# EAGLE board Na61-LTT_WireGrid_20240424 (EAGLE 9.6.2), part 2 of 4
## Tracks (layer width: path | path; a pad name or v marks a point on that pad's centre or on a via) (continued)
S$1547 (continued)
  Bottom 0.152: 49.8,31 49.4,31
S$1548
  Bottom 0.152: 49.4,31 48.4,32
S$1549
  Bottom 0.152: 47.8,31 46.8,32
S$1550
  Bottom 0.152: 45.8,31 45.2,31.6
S$1551
  Bottom 0.152: 45.2,31.6 45.2,32
S$1552
  Bottom 0.152: 43.8,31 43.6,31.2
S$1553
  Bottom 0.152: 43.6,31.2 43.6,32
S$1554
  Bottom 0.152: 41.8,31 42,31.2
S$1555
  Bottom 0.152: 42,31.2 42,32
S$1556
  Bottom 0.152: 39.8,31 40.4,31.6
S$1557
  Bottom 0.152: 40.4,31.6 40.4,32
S$1558
  Bottom 0.152: 37.8,31 38.8,32
S$1559
  Bottom 0.152: 35.8,31 36.2,31
S$1560
  Bottom 0.152: 36.2,31 37.2,32
S$1561
  Bottom 0.152: 33.8,31 34.6,31
S$1562
  Bottom 0.152: 34.6,31 35.6,32
S$1563
  Bottom 0.152: 40.8,35 41.2,35.4
S$1564
  Bottom 0.152: 41.2,35.4 41.2,36
S$1565
  Bottom 0.152: 38.8,35 39.6,35.8
S$1566
  Bottom 0.152: 39.6,35.8 39.6,36
S$1567
  Bottom 0.152: 36.8,35 37,35
S$1568
  Bottom 0.152: 37,35 38,36
S$1569
  Bottom 0.152: 34.8,35 35.4,35
S$1570
  Bottom 0.152: 35.4,35 36.4,36
S$1571
  Bottom 0.152: 32.8,33 33.8,32
S$1572
  Bottom 0.152: 33.8,32 34.8,32
S$1573
  Bottom 0.152: 34.6,37 34,37
S$1574
  Bottom 0.152: 34,37 33,36
S$1575
  Bottom 0.152: 33,36 32.4,36
S$1576
  Bottom 0.152: 32.6,37 31.6,36
S$1577
  Bottom 0.152: 31.6,36 30.8,36
S$1578
  Bottom 0.152: 30.6,37 29.6,36
S$1579
  Bottom 0.152: 29.6,36 29.2,36
S$1580
  Bottom 0.152: 28.6,37 27.6,36
S$1581
  Bottom 0.152: 26.6,37 26,36.4
S$1582
  Bottom 0.152: 26,36.4 26,36
S$1583
  Bottom 0.152: 35.6,41 34.6,40
S$1584
  Bottom 0.152: 34.6,40 33.2,40
S$1585
  Bottom 0.152: 33.6,41 33.2,41
S$1586
  Bottom 0.152: 33.2,41 32.2,40
S$1587
  Bottom 0.152: 32.2,40 31.6,40
S$1588
  Bottom 0.152: 31.6,41 31,41
S$1589
  Bottom 0.152: 31,41 30,40
S$1590
  Bottom 0.152: 29.6,41 29.4,41
S$1591
  Bottom 0.152: 29.4,41 28.4,40
S$1592
  Bottom 0.152: 27.6,41 26.8,40.2
S$1593
  Bottom 0.152: 26.8,40.2 26.8,40
S$1594
  Bottom 0.152: 34,36 35.2,36
S$1595
  Bottom 0.152: 35.2,36 36.2,37
S$1596
  Bottom 0.152: 36.2,37 36.6,37
S$1597  (2 unrouted)
  Top 0.813: 65,40.5 65,31.5
  Top 1.8: 66,37.5 64,37.5 | 66,40.5 65,40.5 64,40.5 | 66,34.5 64,34.5 | 66,31.5 65,31.5 64,31.5
S$1598
  Top 1.778: -104.08,32.83 -104.08,34.35
S$1599
  Top 1.778: -104.08,37.65 -104.08,39.17
S$1600
  Top 1.778: -99,32.83 -99,34.35
S$1601
  Top 1.778: -99,37.65 -99,39.17
S$1602
  Top 1.778: -93.92,32.83 -93.92,34.35
S$1603
  Top 1.778: -93.92,37.65 -93.92,39.17
S$1604
  Top 1.778: 93.92,32.83 93.92,34.35
S$1605
  Top 1.778: 93.92,37.65 93.92,39.17
S$1606
  Top 1.778: 99,32.83 99,34.35
S$1607
  Top 1.778: 99,37.65 99,39.17
S$1608
  Top 1.778: 104.08,32.83 104.08,34.35
S$1609
  Top 1.778: 104.08,37.65 104.08,39.17
S$1618
  Bottom 0.8: 9.4,48.9 9.4,47.1
S$1619
  Bottom 0.8: 11.4,48.9 11.4,47.1
S$1620
  Bottom 0.8: 8.4,51.1 8.4,52.9
S$1621
  Bottom 0.8: 10.4,51.1 10.4,52.9
S$1622
  Bottom 0.8: 5.4,48.9 5.4,47.1
S$1623
  Bottom 0.8: 7.4,48.9 7.4,47.1
S$1624
  Bottom 0.8: 6.4,51.1 6.4,52.9
S$1625
  Bottom 0.8: 4.4,51.1 4.4,52.9
S$1626
  Bottom 0.8: 3.4,48.9 3.4,47.1
S$1627
  Bottom 0.8: 1.4,48.9 1.4,47.1
S$1628
  Bottom 0.8: 2.4,51.1 2.4,52.9
S$1629
  Bottom 0.8: 0.4,51.1 0.4,52.9
S$1630
  Bottom 0.8: -0.6,48.9 -0.6,47.1
S$1631
  Bottom 0.8: -2.6,48.9 -2.6,47.1
S$1632
  Bottom 0.8: -1.6,51.1 -1.6,52.9
S$1633
  Bottom 0.8: 17.4,48.9 17.4,47.1
S$1634
  Bottom 0.8: 19.4,48.9 19.4,47.1
S$1635
  Bottom 0.8: 16.4,51.1 16.4,52.9
S$1636
  Bottom 0.8: 18.4,51.1 18.4,52.9
S$1637
  Bottom 0.8: 13.4,48.9 13.4,47.1
S$1638
  Bottom 0.8: 15.4,48.9 15.4,47.1
S$1639
  Bottom 0.8: 12.4,51.1 12.4,52.9
S$1640
  Bottom 0.8: 14.4,51.1 14.4,52.9
S$1641
  Bottom 0.8: -7.4,56.9 -7.4,55.1
S$1642
  Bottom 0.8: -5.4,56.9 -5.4,55.1
S$1643
  Bottom 0.8: -8.4,59.1 -8.4,60.9
S$1644
  Bottom 0.8: -6.4,59.1 -6.4,60.9
S$1645
  Bottom 0.8: -11.4,56.9 -11.4,55.1
S$1646
  Bottom 0.8: -9.4,56.9 -9.4,55.1
S$1647
  Bottom 0.8: -10.4,59.1 -10.4,60.9
S$1648
  Bottom 0.8: -12.4,59.1 -12.4,60.9
S$1649
  Bottom 0.8: -13.4,56.9 -13.4,55.1
S$1650
  Bottom 0.8: -15.4,56.9 -15.4,55.1
S$1651
  Bottom 0.8: -14.4,59.1 -14.4,60.9
S$1652
  Bottom 0.8: -16.4,59.1 -16.4,60.9
S$1653
  Bottom 0.8: -17.4,56.9 -17.4,55.1
S$1654
  Bottom 0.8: -19.4,56.9 -19.4,55.1
S$1655
  Bottom 0.8: -18.4,59.1 -18.4,60.9
S$1656
  Bottom 0.8: 0.6,56.9 0.6,55.1
S$1657
  Bottom 0.8: 2.6,56.9 2.6,55.1
S$1658
  Bottom 0.8: -0.4,59.1 -0.4,60.9
S$1659
  Bottom 0.8: 1.6,59.1 1.6,60.9
S$1660
  Bottom 0.8: -3.4,56.9 -3.4,55.1
S$1661
  Bottom 0.8: -1.4,56.9 -1.4,55.1
S$1662
  Bottom 0.8: -4.4,59.1 -4.4,60.9
S$1663
  Bottom 0.8: -2.4,59.1 -2.4,60.9
S$1664
  Bottom 0.8: -24.6,48.9 -24.6,47.1
S$1665
  Bottom 0.8: -22.6,48.9 -22.6,47.1
S$1666
  Bottom 0.8: -25.6,51.1 -25.6,52.9
S$1667
  Bottom 0.8: -23.6,51.1 -23.6,52.9
S$1668
  Bottom 0.8: -28.6,48.9 -28.6,47.1
S$1669
  Bottom 0.8: -26.6,48.9 -26.6,47.1
S$1670
  Bottom 0.8: -27.6,51.1 -27.6,52.9
S$1671
  Bottom 0.8: -29.6,51.1 -29.6,52.9
S$1672
  Bottom 0.8: -30.6,48.9 -30.6,47.1
S$1673
  Bottom 0.8: -32.6,48.9 -32.6,47.1
S$1674
  Bottom 0.8: -31.6,51.1 -31.6,52.9
S$1675
  Bottom 0.8: -33.6,51.1 -33.6,52.9
S$1676
  Bottom 0.8: -34.6,48.9 -34.6,47.1
S$1677
  Bottom 0.8: -36.6,48.9 -36.6,47.1
S$1678
  Bottom 0.8: -35.6,51.1 -35.6,52.9
S$1679
  Bottom 0.8: -16.6,48.9 -16.6,47.1
S$1680
  Bottom 0.8: -14.6,48.9 -14.6,47.1
S$1681
  Bottom 0.8: -17.6,51.1 -17.6,52.9
S$1682
  Bottom 0.8: -15.6,51.1 -15.6,52.9
S$1683
  Bottom 0.8: -20.6,48.9 -20.6,47.1
S$1684
  Bottom 0.8: -18.6,48.9 -18.6,47.1
S$1685
  Bottom 0.8: -21.6,51.1 -21.6,52.9
S$1686
  Bottom 0.8: -19.6,51.1 -19.6,52.9
S$1687
  Bottom 0.8: 26.6,56.9 26.6,55.1
S$1688
  Bottom 0.8: 28.6,56.9 28.6,55.1
S$1689
  Bottom 0.8: 25.6,59.1 25.6,60.9
S$1690
  Bottom 0.8: 27.6,59.1 27.6,60.9
S$1691
  Bottom 0.8: 22.6,56.9 22.6,55.1
S$1692
  Bottom 0.8: 24.6,56.9 24.6,55.1
S$1693
  Bottom 0.8: 23.6,59.1 23.6,60.9
S$1694
  Bottom 0.8: 21.6,59.1 21.6,60.9
S$1695
  Bottom 0.8: 20.6,56.9 20.6,55.1
S$1696
  Bottom 0.8: 18.6,56.9 18.6,55.1
S$1697
  Bottom 0.8: 19.6,59.1 19.6,60.9
S$1698
  Bottom 0.8: 17.6,59.1 17.6,60.9
S$1699
  Bottom 0.8: 16.6,56.9 16.6,55.1
S$1700
  Bottom 0.8: 14.6,56.9 14.6,55.1
S$1701
  Bottom 0.8: 15.6,59.1 15.6,60.9
S$1702
  Bottom 0.8: 34.6,56.9 34.6,55.1
S$1703
  Bottom 0.8: 36.6,56.9 36.6,55.1
S$1704
  Bottom 0.8: 33.6,59.1 33.6,60.9
S$1705
  Bottom 0.8: 35.6,59.1 35.6,60.9
S$1706
  Bottom 0.8: 30.6,56.9 30.6,55.1
S$1707
  Bottom 0.8: 32.6,56.9 32.6,55.1
S$1708
  Bottom 0.8: 29.6,59.1 29.6,60.9
S$1709
  Bottom 0.8: 31.6,59.1 31.6,60.9
S$1710
  Bottom 0.8: -41.8,56.9 -41.8,55.1
S$1711
  Bottom 0.8: -39.8,56.9 -39.8,55.1
S$1712
  Bottom 0.8: -42.8,59.1 -42.8,60.9
S$1713
  Bottom 0.8: -40.8,59.1 -40.8,60.9
S$1714
  Bottom 0.8: -45.8,56.9 -45.8,55.1
S$1715
  Bottom 0.8: -43.8,56.9 -43.8,55.1
S$1716
  Bottom 0.8: -44.8,59.1 -44.8,60.9
S$1717
  Bottom 0.8: -46.8,59.1 -46.8,60.9
S$1718
  Bottom 0.8: -47.8,56.9 -47.8,55.1
S$1719
  Bottom 0.8: -49.8,56.9 -49.8,55.1
S$1720
  Bottom 0.8: -48.8,59.1 -48.8,60.9
S$1721
  Bottom 0.8: -50.8,59.1 -50.8,60.9
S$1722
  Bottom 0.8: -51.8,56.9 -51.8,55.1
S$1723
  Bottom 0.8: -53.8,56.9 -53.8,55.1
S$1724
  Bottom 0.8: -52.8,59.1 -52.8,60.9
S$1725
  Bottom 0.8: -33.8,56.9 -33.8,55.1
S$1726
  Bottom 0.8: -31.8,56.9 -31.8,55.1
S$1727
  Bottom 0.8: -34.8,59.1 -34.8,60.9
S$1728
  Bottom 0.8: -32.8,59.1 -32.8,60.9
S$1729
  Bottom 0.8: -37.8,56.9 -37.8,55.1
S$1730
  Bottom 0.8: -35.8,56.9 -35.8,55.1
S$1731
  Bottom 0.8: -38.8,59.1 -38.8,60.9
S$1732
  Bottom 0.8: -36.8,59.1 -36.8,60.9
S$1733
  Bottom 0.8: 43.8,48.9 43.8,47.1
S$1734
  Bottom 0.8: 45.8,48.9 45.8,47.1
S$1735
  Bottom 0.8: 42.8,51.1 42.8,52.9
S$1736
  Bottom 0.8: 44.8,51.1 44.8,52.9
S$1737
  Bottom 0.8: 39.8,48.9 39.8,47.1
S$1738
  Bottom 0.8: 41.8,48.9 41.8,47.1
S$1739
  Bottom 0.8: 40.8,51.1 40.8,52.9
S$1740
  Bottom 0.8: 38.8,51.1 38.8,52.9
S$1741
  Bottom 0.8: 37.8,48.9 37.8,47.1
S$1742
  Bottom 0.8: 35.8,48.9 35.8,47.1
S$1743
  Bottom 0.8: 36.8,51.1 36.8,52.9
S$1744
  Bottom 0.8: 34.8,51.1 34.8,52.9
S$1745
  Bottom 0.8: 33.8,48.9 33.8,47.1
S$1746
  Bottom 0.8: 31.8,48.9 31.8,47.1
S$1747
  Bottom 0.8: 32.8,51.1 32.8,52.9
S$1748
  Bottom 0.8: 51.8,48.9 51.8,47.1
S$1749
  Bottom 0.8: 53.8,48.9 53.8,47.1
S$1750
  Bottom 0.8: 50.8,51.1 50.8,52.9
S$1751
  Bottom 0.8: 52.8,51.1 52.8,52.9
S$1752
  Bottom 0.8: 47.8,48.9 47.8,47.1
S$1753
  Bottom 0.8: 49.8,48.9 49.8,47.1
S$1754
  Bottom 0.8: 46.8,51.1 46.8,52.9
S$1755
  Bottom 0.8: 48.8,51.1 48.8,52.9
S$1884
  Bottom 0.152: -52.8,59 -51.8,58
S$1885
  Bottom 0.152: -51.8,58 -50.8,58
S$1886
  Bottom 0.152: -50.8,59 -50.2,59
S$1887
  Bottom 0.152: -50.2,59 -49.2,58
S$1888
  Bottom 0.152: -48.8,59 -48.6,59
S$1889
  Bottom 0.152: -48.6,59 -47.6,58
S$1890
  Bottom 0.152: -46.8,59 -46,58.2
S$1891
  Bottom 0.152: -46,58.2 -46,58
S$1892
  Bottom 0.152: -44.8,59 -44.4,58.6
S$1893
  Bottom 0.152: -44.4,58.6 -44.4,58
S$1894
  Bottom 0.152: -42.8,59 -42.8,58
S$1895
  Bottom 0.152: -40.8,59 -41.2,58.6
S$1896
  Bottom 0.152: -41.2,58.6 -41.2,58
S$1897
  Bottom 0.152: -38.8,59 -39.6,58.2
S$1898
  Bottom 0.152: -39.6,58.2 -39.6,58
S$1899
  Bottom 0.152: -36.8,59 -37,59
S$1900
  Bottom 0.152: -37,59 -38,58
S$1901
  Bottom 0.152: -34.8,59 -35.4,59
S$1902
  Bottom 0.152: -35.4,59 -36.4,58
S$1903
  Bottom 0.152: -32.8,59 -33.8,58
S$1904
  Bottom 0.152: -33.8,58 -34.8,58
S$1905
  Bottom 0.152: -51.8,55 -50.8,54
S$1906
  Bottom 0.152: -50.8,54 -50,54
S$1907
  Bottom 0.152: -49.8,55 -48.8,54
S$1908
  Bottom 0.152: -48.8,54 -48.4,54
S$1909
  Bottom 0.152: -47.8,55 -46.8,54
S$1910
  Bottom 0.152: -45.8,55 -45.2,54.4
S$1911
  Bottom 0.152: -45.2,54.4 -45.2,54
S$1912
  Bottom 0.152: -43.8,55 -43.6,54.8
S$1913
  Bottom 0.152: -43.6,54.8 -43.6,54
S$1914
  Bottom 0.152: -41.8,55 -42,54.8
S$1915
  Bottom 0.152: -42,54.8 -42,54
S$1916
  Bottom 0.152: -39.8,55 -40.4,54.4
S$1917
  Bottom 0.152: -40.4,54.4 -40.4,54
S$1918
  Bottom 0.152: -37.8,55 -38.8,54
S$1919
  Bottom 0.152: -35.8,55 -36.8,54
S$1920
  Bottom 0.152: -36.8,54 -37.2,54
S$1921
  Bottom 0.152: -33.8,55 -34.8,54
S$1922
  Bottom 0.152: -34.8,54 -35.6,54
S$1923
  Bottom 0.152: -36.6,49 -35.6,50
S$1924
  Bottom 0.152: -35.6,50 -34,50
S$1925
  Bottom 0.152: -34.6,49 -33.8,49
S$1926
  Bottom 0.152: -33.8,49 -32.8,50
S$1927
  Bottom 0.152: -32.8,50 -32.4,50
S$1928
  Bottom 0.152: -32.6,49 -31.8,49
S$1929
  Bottom 0.152: -31.8,49 -30.8,50
S$1930
  Bottom 0.152: -30.6,49 -30.2,49
S$1931
  Bottom 0.152: -30.2,49 -29.2,50
S$1932
  Bottom 0.152: -28.6,49 -27.6,50
S$1933
  Bottom 0.152: -26.6,49 -26,49.6
S$1934
  Bottom 0.152: -26,49.6 -26,50
S$1935
  Bottom 0.152: -35.6,53 -35,53
S$1936
  Bottom 0.152: -35,53 -34,54
S$1937
  Bottom 0.152: -34,54 -33.2,54
S$1938
  Bottom 0.152: -33.6,53 -33,53
S$1939
  Bottom 0.152: -33,53 -32,54
S$1940
  Bottom 0.152: -32,54 -31.6,54
S$1941
  Bottom 0.152: -31.6,53 -31,53
S$1942
  Bottom 0.152: -31,53 -30,54
S$1943
  Bottom 0.152: -29.6,53 -29.4,53
S$1944
  Bottom 0.152: -29.4,53 -28.4,54
S$1945
  Bottom 0.152: -27.6,53 -26.8,53.8
S$1946
  Bottom 0.152: -26.8,53.8 -26.8,54
S$1947
  Bottom 0.152: 1.6,59 0.6,58
S$1948
  Bottom 0.152: 0.6,58 -0.4,58
S$1949
  Bottom 0.152: -0.4,59 -1,59
S$1950
  Bottom 0.152: -1,59 -2,58
S$1951
  Bottom 0.152: -2.4,59 -2.6,59
S$1952
  Bottom 0.152: -2.6,59 -3.6,58
S$1953
  Bottom 0.152: -4.4,59 -5.2,58.2
S$1954
  Bottom 0.152: -5.2,58.2 -5.2,58
S$1955
  Bottom 0.152: -6.4,59 -6.8,58.6
S$1956
  Bottom 0.152: -6.8,58.6 -6.8,58
S$1957
  Bottom 0.152: -8.4,59 -8.4,58
S$1958
  Bottom 0.152: -10.4,59 -10,58.6
S$1959
  Bottom 0.152: -10,58.6 -10,58
S$1960
  Bottom 0.152: -12.4,59 -11.6,58.2
S$1961
  Bottom 0.152: -11.6,58.2 -11.6,58
S$1962
  Bottom 0.152: -14.4,59 -14.2,59
S$1963
  Bottom 0.152: -14.2,59 -13.2,58
S$1964
  Bottom 0.152: -16.4,59 -15.8,59
S$1965
  Bottom 0.152: -15.8,59 -14.8,58
S$1966
  Bottom 0.152: -18.4,59 -17.4,58
S$1967
  Bottom 0.152: -17.4,58 -16.4,58
S$1968
  Bottom 0.152: 0.6,55 -0.4,54
S$1969
  Bottom 0.152: -0.4,54 -1.2,54
S$1970
  Bottom 0.152: -1.4,55 -2.4,54
S$1971
  Bottom 0.152: -2.4,54 -2.8,54
S$1972
  Bottom 0.152: -3.4,55 -4.4,54
S$1973
  Bottom 0.152: -5.4,55 -6,54.4
S$1974
  Bottom 0.152: -6,54.4 -6,54
S$1975
  Bottom 0.152: -7.4,55 -7.6,54.8
S$1976
  Bottom 0.152: -7.6,54.8 -7.6,54
S$1977
  Bottom 0.152: -9.4,55 -9.2,54.8
S$1978
  Bottom 0.152: -9.2,54.8 -9.2,54
S$1979
  Bottom 0.152: -11.4,55 -10.8,54.4
S$1980
  Bottom 0.152: -10.8,54.4 -10.8,54
S$1981
  Bottom 0.152: -13.4,55 -12.4,54
S$1982
  Bottom 0.152: -15.4,55 -14.4,54
S$1983
  Bottom 0.152: -14.4,54 -14,54
S$1984
  Bottom 0.152: -17.4,55 -16.4,54
S$1985
  Bottom 0.152: -16.4,54 -15.6,54
S$1986
  Bottom 0.152: -14.6,49 -15.6,50
S$1987
  Bottom 0.152: -15.6,50 -17.2,50
S$1988
  Bottom 0.152: -16.6,49 -17.4,49
S$1989
  Bottom 0.152: -17.4,49 -18.4,50
S$1990
  Bottom 0.152: -18.4,50 -18.8,50
S$1991
  Bottom 0.152: -18.6,49 -19.4,49
S$1992
  Bottom 0.152: -19.4,49 -20.4,50
S$1993
  Bottom 0.152: -20.6,49 -21,49
S$1994
  Bottom 0.152: -21,49 -22,50
S$1995
  Bottom 0.152: -22.6,49 -23.6,50
S$1996
  Bottom 0.152: -24.6,49 -25.2,49.6
S$1997
  Bottom 0.152: -25.2,49.6 -25.2,50
S$1998
  Bottom 0.152: -15.6,53 -16.2,53
S$1999
  Bottom 0.152: -16.2,53 -17.2,54
S$2000
  Bottom 0.152: -17.2,54 -18,54
S$2001
  Bottom 0.152: -17.6,53 -18.2,53
S$2002
  Bottom 0.152: -18.2,53 -19.2,54
S$2003
  Bottom 0.152: -19.2,54 -19.6,54
S$2004
  Bottom 0.152: -19.6,53 -20.2,53
S$2005
  Bottom 0.152: -20.2,53 -21.2,54
S$2006
  Bottom 0.152: -21.6,53 -21.8,53
S$2007
  Bottom 0.152: -21.8,53 -22.8,54
S$2008
  Bottom 0.152: -23.6,53 -24.4,53.8
S$2009
  Bottom 0.152: -24.4,53.8 -24.4,54
S$2010
  Bottom 0.152: 0.4,53 1,53
S$2011
  Bottom 0.152: 1,53 2,54
S$2012
  Bottom 0.152: 2.4,53 2.6,53
S$2013
  Bottom 0.152: 2.6,53 3.6,54
S$2014
  Bottom 0.152: 4.4,53 5.2,53.8
S$2015
  Bottom 0.152: 5.2,53.8 5.2,54
S$2016
  Bottom 0.152: 6.4,53 6.8,53.4
S$2017
  Bottom 0.152: 6.8,53.4 6.8,54
S$2018
  Bottom 0.152: 8.4,53 8.4,54
S$2019
  Bottom 0.152: -1.6,53 -0.6,53
S$2020
  Bottom 0.152: -0.6,53 0.4,54
S$2021
  Bottom 0.152: -0.6,49 0.4,50
S$2022
  Bottom 0.152: 0.4,50 1.2,50
S$2023
  Bottom 0.152: 1.4,49 1.8,49
S$2024
  Bottom 0.152: 1.8,49 2.8,50
S$2025
  Bottom 0.152: 3.4,49 4.4,50
S$2026
  Bottom 0.152: 5.4,49 6,49.6
S$2027
  Bottom 0.152: 6,49.6 6,50
S$2028
  Bottom 0.152: 7.4,49 7.6,49.2
S$2029
  Bottom 0.152: 7.6,49.2 7.6,50
S$2030
  Bottom 0.152: 9.4,49 9.2,49.2
S$2031
  Bottom 0.152: 9.2,49.2 9.2,50
S$2032
  Bottom 0.152: 11.4,49 10.8,49.6
S$2033
  Bottom 0.152: 10.8,49.6 10.8,50
S$2034
  Bottom 0.152: 13.4,49 12.4,50
S$2035
  Bottom 0.152: 15.4,49 15,49
S$2036
  Bottom 0.152: 15,49 14,50
S$2037
  Bottom 0.152: 17.4,49 16.6,49
S$2038
  Bottom 0.152: 16.6,49 15.6,50
S$2039
  Bottom 0.152: 10.4,53 10,53.4
S$2040
  Bottom 0.152: 10,53.4 10,54
S$2041
  Bottom 0.152: 12.4,53 11.6,53.8
S$2042
  Bottom 0.152: 11.6,53.8 11.6,54
S$2043
  Bottom 0.152: 14.4,53 14.2,53
S$2044
  Bottom 0.152: 14.2,53 13.2,54
S$2045
  Bottom 0.152: 16.4,53 15.8,53
S$2046
  Bottom 0.152: 15.8,53 14.8,54
S$2047
  Bottom 0.152: 18.4,51 17.4,50
S$2048
  Bottom 0.152: 17.4,50 16.4,50
S$2049
  Bottom 0.152: 16.6,55 17.2,55
S$2050
  Bottom 0.152: 17.2,55 18.2,54
S$2051
  Bottom 0.152: 18.2,54 18.8,54
S$2052
  Bottom 0.152: 18.6,55 19.6,54
S$2053
  Bottom 0.152: 19.6,54 20.4,54
S$2054
  Bottom 0.152: 20.6,55 21.6,54
S$2055
  Bottom 0.152: 21.6,54 22,54
S$2056
  Bottom 0.152: 22.6,55 23.6,54
S$2057
  Bottom 0.152: 24.6,55 25.2,54.4
S$2058
  Bottom 0.152: 25.2,54.4 25.2,54
S$2059
  Bottom 0.152: 15.6,59 16.6,58
S$2060
  Bottom 0.152: 16.6,58 18,58
S$2061
  Bottom 0.152: 17.6,59 18,59
S$2062
  Bottom 0.152: 18,59 19,58
S$2063
  Bottom 0.152: 19,58 19.6,58
S$2064
  Bottom 0.152: 19.6,59 20.2,59
S$2065
  Bottom 0.152: 20.2,59 21.2,58
S$2066
  Bottom 0.152: 21.6,59 21.8,59
S$2067
  Bottom 0.152: 21.8,59 22.8,58
S$2068
  Bottom 0.152: 23.6,59 24.4,58.2
S$2069
  Bottom 0.152: 24.4,58.2 24.4,58
S$2070
  Bottom 0.152: 17.2,54 16,54
S$2071
  Bottom 0.152: 16,54 15,55
S$2072
  Bottom 0.152: 15,55 14.6,55
S$2073
  Bottom 0.152: 50.8,53 50.2,53
S$2074
  Bottom 0.152: 50.2,53 49.2,54
S$2075
  Bottom 0.152: 48.8,53 48.6,53
S$2076
  Bottom 0.152: 48.6,53 47.6,54
S$2077
  Bottom 0.152: 46.8,53 46,53.8
S$2078
  Bottom 0.152: 46,53.8 46,54
S$2079
  Bottom 0.152: 44.8,53 44.4,53.4
S$2080
  Bottom 0.152: 44.4,53.4 44.4,54
S$2081
  Bottom 0.152: 42.8,53 42.8,54
S$2082
  Bottom 0.152: 52.8,53 51.8,53
S$2083
  Bottom 0.152: 51.8,53 50.8,54
S$2084
  Bottom 0.152: 51.8,49 50.8,50
S$2085
  Bottom 0.152: 50.8,50 50,50
S$2086
  Bottom 0.152: 49.8,49 49.4,49
S$2087
  Bottom 0.152: 49.4,49 48.4,50
S$2088
  Bottom 0.152: 47.8,49 46.8,50
S$2089
  Bottom 0.152: 45.8,49 45.2,49.6
S$2090
  Bottom 0.152: 45.2,49.6 45.2,50
S$2091
  Bottom 0.152: 43.8,49 43.6,49.2
S$2092
  Bottom 0.152: 43.6,49.2 43.6,50
S$2093
  Bottom 0.152: 41.8,49 42,49.2
S$2094
  Bottom 0.152: 42,49.2 42,50
S$2095
  Bottom 0.152: 39.8,49 40.4,49.6
S$2096
  Bottom 0.152: 40.4,49.6 40.4,50
S$2097
  Bottom 0.152: 37.8,49 38.8,50
S$2098
  Bottom 0.152: 35.8,49 36.2,49
S$2099
  Bottom 0.152: 36.2,49 37.2,50
S$2100
  Bottom 0.152: 33.8,49 34.6,49
S$2101
  Bottom 0.152: 34.6,49 35.6,50
S$2102
  Bottom 0.152: 40.8,53 41.2,53.4
S$2103
  Bottom 0.152: 41.2,53.4 41.2,54
S$2104
  Bottom 0.152: 38.8,53 39.6,53.8
S$2105
  Bottom 0.152: 39.6,53.8 39.6,54
S$2106
  Bottom 0.152: 36.8,53 37,53
S$2107
  Bottom 0.152: 37,53 38,54
S$2108
  Bottom 0.152: 34.8,53 35.4,53
S$2109
  Bottom 0.152: 35.4,53 36.4,54
S$2110
  Bottom 0.152: 32.8,51 33.8,50
S$2111
  Bottom 0.152: 33.8,50 34.8,50
S$2112
  Bottom 0.152: 34.6,55 34,55
S$2113
  Bottom 0.152: 34,55 33,54
S$2114
  Bottom 0.152: 33,54 32.4,54
S$2115
  Bottom 0.152: 32.6,55 31.6,54
S$2116
  Bottom 0.152: 31.6,54 30.8,54
S$2117
  Bottom 0.152: 30.6,55 29.6,54
S$2118
  Bottom 0.152: 29.6,54 29.2,54
S$2119
  Bottom 0.152: 28.6,55 27.6,54
S$2120
  Bottom 0.152: 26.6,55 26,54.4
S$2121
  Bottom 0.152: 26,54.4 26,54
S$2122
  Bottom 0.152: 35.6,59 34.6,58
S$2123
  Bottom 0.152: 34.6,58 33.2,58
S$2124
  Bottom 0.152: 33.6,59 33.2,59
S$2125
  Bottom 0.152: 33.2,59 32.2,58
S$2126
  Bottom 0.152: 32.2,58 31.6,58
S$2127
  Bottom 0.152: 31.6,59 31,59
S$2128
  Bottom 0.152: 31,59 30,58
S$2129
  Bottom 0.152: 29.6,59 29.4,59
S$2130
  Bottom 0.152: 29.4,59 28.4,58
S$2131
  Bottom 0.152: 27.6,59 26.8,58.2
S$2132
  Bottom 0.152: 26.8,58.2 26.8,58
S$2133
  Bottom 0.152: 34,54 35.2,54
S$2134
  Bottom 0.152: 35.2,54 36.2,55
S$2135
  Bottom 0.152: 36.2,55 36.6,55
S$2136  (2 unrouted)
  Top 0.813: 65,58.5 65,49.5
  Top 1.8: 66,55.5 64,55.5 | 66,58.5 65,58.5 64,58.5 | 66,52.5 64,52.5 | 66,49.5 65,49.5 64,49.5
S$2137
  Top 1.778: -104.08,50.83 -104.08,52.35
S$2138
  Top 1.778: -104.08,55.65 -104.08,57.17
S$2139
  Top 1.778: -99,50.83 -99,52.35
S$2140
  Top 1.778: -99,55.65 -99,57.17
S$2141
  Top 1.778: -93.92,50.83 -93.92,52.35
S$2142
  Top 1.778: -93.92,55.65 -93.92,57.17
S$2143
  Top 1.778: 93.92,50.83 93.92,52.35
S$2144
  Top 1.778: 93.92,55.65 93.92,57.17
S$2145
  Top 1.778: 99,50.83 99,52.35
S$2146
  Top 1.778: 99,55.65 99,57.17
S$2147
  Top 1.778: 104.08,50.83 104.08,52.35
S$2148
  Top 1.778: 104.08,55.65 104.08,57.17
S$2157
  Bottom 0.8: 9.4,66.9 9.4,65.1
S$2158
  Bottom 0.8: 11.4,66.9 11.4,65.1
S$2159
  Bottom 0.8: 8.4,69.1 8.4,70.9
S$2160
  Bottom 0.8: 10.4,69.1 10.4,70.9
S$2161
  Bottom 0.8: 5.4,66.9 5.4,65.1
S$2162
  Bottom 0.8: 7.4,66.9 7.4,65.1
S$2163
  Bottom 0.8: 6.4,69.1 6.4,70.9
S$2164
  Bottom 0.8: 4.4,69.1 4.4,70.9
S$2165
  Bottom 0.8: 3.4,66.9 3.4,65.1
S$2166
  Bottom 0.8: 1.4,66.9 1.4,65.1
S$2167
  Bottom 0.8: 2.4,69.1 2.4,70.9
S$2168
  Bottom 0.8: 0.4,69.1 0.4,70.9
S$2169
  Bottom 0.8: -0.6,66.9 -0.6,65.1
S$2170
  Bottom 0.8: -2.6,66.9 -2.6,65.1
S$2171
  Bottom 0.8: -1.6,69.1 -1.6,70.9
S$2172
  Bottom 0.8: 17.4,66.9 17.4,65.1
S$2173
  Bottom 0.8: 19.4,66.9 19.4,65.1
S$2174
  Bottom 0.8: 16.4,69.1 16.4,70.9
S$2175
  Bottom 0.8: 18.4,69.1 18.4,70.9
S$2176
  Bottom 0.8: 13.4,66.9 13.4,65.1
S$2177
  Bottom 0.8: 15.4,66.9 15.4,65.1
S$2178
  Bottom 0.8: 12.4,69.1 12.4,70.9
S$2179
  Bottom 0.8: 14.4,69.1 14.4,70.9
S$2180
  Bottom 0.8: -7.4,74.9 -7.4,73.1
S$2181
  Bottom 0.8: -5.4,74.9 -5.4,73.1
S$2182
  Bottom 0.8: -8.4,77.1 -8.4,78.9
S$2183
  Bottom 0.8: -6.4,77.1 -6.4,78.9
S$2184
  Bottom 0.8: -11.4,74.9 -11.4,73.1
S$2185
  Bottom 0.8: -9.4,74.9 -9.4,73.1
S$2186
  Bottom 0.8: -10.4,77.1 -10.4,78.9
S$2187
  Bottom 0.8: -12.4,77.1 -12.4,78.9
S$2188
  Bottom 0.8: -13.4,74.9 -13.4,73.1
S$2189
  Bottom 0.8: -15.4,74.9 -15.4,73.1
S$2190
  Bottom 0.8: -14.4,77.1 -14.4,78.9
S$2191
  Bottom 0.8: -16.4,77.1 -16.4,78.9
S$2192
  Bottom 0.8: -17.4,74.9 -17.4,73.1
S$2193
  Bottom 0.8: -19.4,74.9 -19.4,73.1
S$2194
  Bottom 0.8: -18.4,77.1 -18.4,78.9
S$2195
  Bottom 0.8: 0.6,74.9 0.6,73.1
S$2196
  Bottom 0.8: 2.6,74.9 2.6,73.1
S$2197
  Bottom 0.8: -0.4,77.1 -0.4,78.9
S$2198
  Bottom 0.8: 1.6,77.1 1.6,78.9
S$2199
  Bottom 0.8: -3.4,74.9 -3.4,73.1
S$2200
  Bottom 0.8: -1.4,74.9 -1.4,73.1
S$2201
  Bottom 0.8: -4.4,77.1 -4.4,78.9
S$2202
  Bottom 0.8: -2.4,77.1 -2.4,78.9
S$2203
  Bottom 0.8: -24.6,66.9 -24.6,65.1
S$2204
  Bottom 0.8: -22.6,66.9 -22.6,65.1
S$2205
  Bottom 0.8: -25.6,69.1 -25.6,70.9
S$2206
  Bottom 0.8: -23.6,69.1 -23.6,70.9
S$2207
  Bottom 0.8: -28.6,66.9 -28.6,65.1
S$2208
  Bottom 0.8: -26.6,66.9 -26.6,65.1
S$2209
  Bottom 0.8: -27.6,69.1 -27.6,70.9
S$2210
  Bottom 0.8: -29.6,69.1 -29.6,70.9
S$2211
  Bottom 0.8: -30.6,66.9 -30.6,65.1
S$2212
  Bottom 0.8: -32.6,66.9 -32.6,65.1
S$2213
  Bottom 0.8: -31.6,69.1 -31.6,70.9
S$2214
  Bottom 0.8: -33.6,69.1 -33.6,70.9
S$2215
  Bottom 0.8: -34.6,66.9 -34.6,65.1
S$2216
  Bottom 0.8: -36.6,66.9 -36.6,65.1
S$2217
  Bottom 0.8: -35.6,69.1 -35.6,70.9
S$2218
  Bottom 0.8: -16.6,66.9 -16.6,65.1
S$2219
  Bottom 0.8: -14.6,66.9 -14.6,65.1
S$2220
  Bottom 0.8: -17.6,69.1 -17.6,70.9
S$2221
  Bottom 0.8: -15.6,69.1 -15.6,70.9
S$2222
  Bottom 0.8: -20.6,66.9 -20.6,65.1
S$2223
  Bottom 0.8: -18.6,66.9 -18.6,65.1
S$2224
  Bottom 0.8: -21.6,69.1 -21.6,70.9
S$2225
  Bottom 0.8: -19.6,69.1 -19.6,70.9
S$2226
  Bottom 0.8: 26.6,74.9 26.6,73.1
S$2227
  Bottom 0.8: 28.6,74.9 28.6,73.1
S$2228
  Bottom 0.8: 25.6,77.1 25.6,78.9
S$2229
  Bottom 0.8: 27.6,77.1 27.6,78.9
S$2230
  Bottom 0.8: 22.6,74.9 22.6,73.1
S$2231
  Bottom 0.8: 24.6,74.9 24.6,73.1
S$2232
  Bottom 0.8: 23.6,77.1 23.6,78.9
S$2233
  Bottom 0.8: 21.6,77.1 21.6,78.9
S$2234
  Bottom 0.8: 20.6,74.9 20.6,73.1
S$2235
  Bottom 0.8: 18.6,74.9 18.6,73.1
S$2236
  Bottom 0.8: 19.6,77.1 19.6,78.9
S$2237
  Bottom 0.8: 17.6,77.1 17.6,78.9
S$2238
  Bottom 0.8: 16.6,74.9 16.6,73.1
S$2239
  Bottom 0.8: 14.6,74.9 14.6,73.1
S$2240
  Bottom 0.8: 15.6,77.1 15.6,78.9
S$2241
  Bottom 0.8: 34.6,74.9 34.6,73.1
S$2242
  Bottom 0.8: 36.6,74.9 36.6,73.1
S$2243
  Bottom 0.8: 33.6,77.1 33.6,78.9
S$2244
  Bottom 0.8: 35.6,77.1 35.6,78.9
S$2245
  Bottom 0.8: 30.6,74.9 30.6,73.1
S$2246
  Bottom 0.8: 32.6,74.9 32.6,73.1
S$2247
  Bottom 0.8: 29.6,77.1 29.6,78.9
S$2248
  Bottom 0.8: 31.6,77.1 31.6,78.9
S$2249
  Bottom 0.8: -41.8,74.9 -41.8,73.1
S$2250
  Bottom 0.8: -39.8,74.9 -39.8,73.1
S$2251
  Bottom 0.8: -42.8,77.1 -42.8,78.9
S$2252
  Bottom 0.8: -40.8,77.1 -40.8,78.9
S$2253
  Bottom 0.8: -45.8,74.9 -45.8,73.1
S$2254
  Bottom 0.8: -43.8,74.9 -43.8,73.1
S$2255
  Bottom 0.8: -44.8,77.1 -44.8,78.9
S$2256
  Bottom 0.8: -46.8,77.1 -46.8,78.9
S$2257
  Bottom 0.8: -47.8,74.9 -47.8,73.1
S$2258
  Bottom 0.8: -49.8,74.9 -49.8,73.1
S$2259
  Bottom 0.8: -48.8,77.1 -48.8,78.9
S$2260
  Bottom 0.8: -50.8,77.1 -50.8,78.9
S$2261
  Bottom 0.8: -51.8,74.9 -51.8,73.1
S$2262
  Bottom 0.8: -53.8,74.9 -53.8,73.1
S$2263
  Bottom 0.8: -52.8,77.1 -52.8,78.9
S$2264
  Bottom 0.8: -33.8,74.9 -33.8,73.1
S$2265
  Bottom 0.8: -31.8,74.9 -31.8,73.1
S$2266
  Bottom 0.8: -34.8,77.1 -34.8,78.9
S$2267
  Bottom 0.8: -32.8,77.1 -32.8,78.9
S$2268
  Bottom 0.8: -37.8,74.9 -37.8,73.1
S$2269
  Bottom 0.8: -35.8,74.9 -35.8,73.1
S$2270
  Bottom 0.8: -38.8,77.1 -38.8,78.9
S$2271
  Bottom 0.8: -36.8,77.1 -36.8,78.9
S$2272
  Bottom 0.8: 43.8,66.9 43.8,65.1
S$2273
  Bottom 0.8: 45.8,66.9 45.8,65.1
S$2274
  Bottom 0.8: 42.8,69.1 42.8,70.9
S$2275
  Bottom 0.8: 44.8,69.1 44.8,70.9
S$2276
  Bottom 0.8: 39.8,66.9 39.8,65.1
S$2277
  Bottom 0.8: 41.8,66.9 41.8,65.1
S$2278
  Bottom 0.8: 40.8,69.1 40.8,70.9
S$2279
  Bottom 0.8: 38.8,69.1 38.8,70.9
S$2280
  Bottom 0.8: 37.8,66.9 37.8,65.1
S$2281
  Bottom 0.8: 35.8,66.9 35.8,65.1
S$2282
  Bottom 0.8: 36.8,69.1 36.8,70.9
S$2283
  Bottom 0.8: 34.8,69.1 34.8,70.9
S$2284
  Bottom 0.8: 33.8,66.9 33.8,65.1
S$2285
  Bottom 0.8: 31.8,66.9 31.8,65.1
S$2286
  Bottom 0.8: 32.8,69.1 32.8,70.9
S$2287
  Bottom 0.8: 51.8,66.9 51.8,65.1
S$2288
  Bottom 0.8: 53.8,66.9 53.8,65.1
S$2289
  Bottom 0.8: 50.8,69.1 50.8,70.9
S$2290
  Bottom 0.8: 52.8,69.1 52.8,70.9
S$2291
  Bottom 0.8: 47.8,66.9 47.8,65.1
S$2292
  Bottom 0.8: 49.8,66.9 49.8,65.1
S$2293
  Bottom 0.8: 46.8,69.1 46.8,70.9
S$2294
  Bottom 0.8: 48.8,69.1 48.8,70.9
S$2423
  Bottom 0.152: -52.8,77 -51.8,76
S$2424
  Bottom 0.152: -51.8,76 -50.8,76
S$2425
  Bottom 0.152: -50.8,77 -50.2,77
S$2426
  Bottom 0.152: -50.2,77 -49.2,76
S$2427
  Bottom 0.152: -48.8,77 -48.6,77
S$2428
  Bottom 0.152: -48.6,77 -47.6,76
S$2429
  Bottom 0.152: -46.8,77 -46,76.2
S$2430
  Bottom 0.152: -46,76.2 -46,76
S$2431
  Bottom 0.152: -44.8,77 -44.4,76.6
S$2432
  Bottom 0.152: -44.4,76.6 -44.4,76
S$2433
  Bottom 0.152: -42.8,77 -42.8,76
S$2434
  Bottom 0.152: -40.8,77 -41.2,76.6
S$2435
  Bottom 0.152: -41.2,76.6 -41.2,76
S$2436
  Bottom 0.152: -38.8,77 -39.6,76.2
S$2437
  Bottom 0.152: -39.6,76.2 -39.6,76
S$2438
  Bottom 0.152: -36.8,77 -37,77
S$2439
  Bottom 0.152: -37,77 -38,76
S$2440
  Bottom 0.152: -34.8,77 -35.4,77
S$2441
  Bottom 0.152: -35.4,77 -36.4,76
S$2442
  Bottom 0.152: -32.8,77 -33.8,76
S$2443
  Bottom 0.152: -33.8,76 -34.8,76
S$2444
  Bottom 0.152: -51.8,73 -50.8,72
S$2445
  Bottom 0.152: -50.8,72 -50,72
S$2446
  Bottom 0.152: -49.8,73 -48.8,72
S$2447
  Bottom 0.152: -48.8,72 -48.4,72
S$2448
  Bottom 0.152: -47.8,73 -46.8,72
S$2449
  Bottom 0.152: -45.8,73 -45.2,72.4
S$2450
  Bottom 0.152: -45.2,72.4 -45.2,72
S$2451
  Bottom 0.152: -43.8,73 -43.6,72.8
S$2452
  Bottom 0.152: -43.6,72.8 -43.6,72
S$2453
  Bottom 0.152: -41.8,73 -42,72.8
S$2454
  Bottom 0.152: -42,72.8 -42,72
S$2455
  Bottom 0.152: -39.8,73 -40.4,72.4
S$2456
  Bottom 0.152: -40.4,72.4 -40.4,72
S$2457
  Bottom 0.152: -37.8,73 -38.8,72
S$2458
  Bottom 0.152: -35.8,73 -36.8,72
S$2459
  Bottom 0.152: -36.8,72 -37.2,72
S$2460
  Bottom 0.152: -33.8,73 -34.8,72
S$2461
  Bottom 0.152: -34.8,72 -35.6,72
S$2462
  Bottom 0.152: -36.6,67 -35.6,68
S$2463
  Bottom 0.152: -35.6,68 -34,68
S$2464
  Bottom 0.152: -34.6,67 -33.8,67
S$2465
  Bottom 0.152: -33.8,67 -32.8,68
S$2466
  Bottom 0.152: -32.8,68 -32.4,68
S$2467
  Bottom 0.152: -32.6,67 -31.8,67
S$2468
  Bottom 0.152: -31.8,67 -30.8,68
S$2469
  Bottom 0.152: -30.6,67 -30.2,67
S$2470
  Bottom 0.152: -30.2,67 -29.2,68
S$2471
  Bottom 0.152: -28.6,67 -27.6,68
S$2472
  Bottom 0.152: -26.6,67 -26,67.6
S$2473
  Bottom 0.152: -26,67.6 -26,68
S$2474
  Bottom 0.152: -35.6,71 -35,71
S$2475
  Bottom 0.152: -35,71 -34,72
S$2476
  Bottom 0.152: -34,72 -33.2,72
S$2477
  Bottom 0.152: -33.6,71 -33,71
S$2478
  Bottom 0.152: -33,71 -32,72
S$2479
  Bottom 0.152: -32,72 -31.6,72
S$2480
  Bottom 0.152: -31.6,71 -31,71
S$2481
  Bottom 0.152: -31,71 -30,72
S$2482
  Bottom 0.152: -29.6,71 -29.4,71
S$2483
  Bottom 0.152: -29.4,71 -28.4,72
S$2484
  Bottom 0.152: -27.6,71 -26.8,71.8
S$2485
  Bottom 0.152: -26.8,71.8 -26.8,72
S$2486
  Bottom 0.152: 1.6,77 0.6,76
S$2487
  Bottom 0.152: 0.6,76 -0.4,76
S$2488
  Bottom 0.152: -0.4,77 -1,77
S$2489
  Bottom 0.152: -1,77 -2,76
S$2490
  Bottom 0.152: -2.4,77 -2.6,77
S$2491
  Bottom 0.152: -2.6,77 -3.6,76
S$2492
  Bottom 0.152: -4.4,77 -5.2,76.2
S$2493
  Bottom 0.152: -5.2,76.2 -5.2,76
S$2494
  Bottom 0.152: -6.4,77 -6.8,76.6
S$2495
  Bottom 0.152: -6.8,76.6 -6.8,76
S$2496
  Bottom 0.152: -8.4,77 -8.4,76
S$2497
  Bottom 0.152: -10.4,77 -10,76.6
S$2498
  Bottom 0.152: -10,76.6 -10,76
S$2499
  Bottom 0.152: -12.4,77 -11.6,76.2
S$2500
  Bottom 0.152: -11.6,76.2 -11.6,76
S$2501
  Bottom 0.152: -14.4,77 -14.2,77
S$2502
  Bottom 0.152: -14.2,77 -13.2,76
S$2503
  Bottom 0.152: -16.4,77 -15.8,77
S$2504
  Bottom 0.152: -15.8,77 -14.8,76
S$2505
  Bottom 0.152: -18.4,77 -17.4,76
S$2506
  Bottom 0.152: -17.4,76 -16.4,76
S$2507
  Bottom 0.152: 0.6,73 -0.4,72
S$2508
  Bottom 0.152: -0.4,72 -1.2,72
S$2509
  Bottom 0.152: -1.4,73 -2.4,72
S$2510
  Bottom 0.152: -2.4,72 -2.8,72
S$2511
  Bottom 0.152: -3.4,73 -4.4,72
S$2512
  Bottom 0.152: -5.4,73 -6,72.4
S$2513
  Bottom 0.152: -6,72.4 -6,72
S$2514
  Bottom 0.152: -7.4,73 -7.6,72.8
S$2515
  Bottom 0.152: -7.6,72.8 -7.6,72
S$2516
  Bottom 0.152: -9.4,73 -9.2,72.8
S$2517
  Bottom 0.152: -9.2,72.8 -9.2,72
S$2518
  Bottom 0.152: -11.4,73 -10.8,72.4
S$2519
  Bottom 0.152: -10.8,72.4 -10.8,72
S$2520
  Bottom 0.152: -13.4,73 -12.4,72
S$2521
  Bottom 0.152: -15.4,73 -14.4,72
S$2522
  Bottom 0.152: -14.4,72 -14,72
S$2523
  Bottom 0.152: -17.4,73 -16.4,72
S$2524
  Bottom 0.152: -16.4,72 -15.6,72
S$2525
  Bottom 0.152: -14.6,67 -15.6,68
S$2526
  Bottom 0.152: -15.6,68 -17.2,68
S$2527
  Bottom 0.152: -16.6,67 -17.4,67
S$2528
  Bottom 0.152: -17.4,67 -18.4,68
S$2529
  Bottom 0.152: -18.4,68 -18.8,68
S$2530
  Bottom 0.152: -18.6,67 -19.4,67
S$2531
  Bottom 0.152: -19.4,67 -20.4,68
S$2532
  Bottom 0.152: -20.6,67 -21,67
S$2533
  Bottom 0.152: -21,67 -22,68
S$2534
  Bottom 0.152: -22.6,67 -23.6,68
S$2535
  Bottom 0.152: -24.6,67 -25.2,67.6
S$2536
  Bottom 0.152: -25.2,67.6 -25.2,68
S$2537
  Bottom 0.152: -15.6,71 -16.2,71
S$2538
  Bottom 0.152: -16.2,71 -17.2,72
S$2539
  Bottom 0.152: -17.2,72 -18,72
S$2540
  Bottom 0.152: -17.6,71 -18.2,71
S$2541
  Bottom 0.152: -18.2,71 -19.2,72
S$2542
  Bottom 0.152: -19.2,72 -19.6,72
S$2543
  Bottom 0.152: -19.6,71 -20.2,71
S$2544
  Bottom 0.152: -20.2,71 -21.2,72
S$2545
  Bottom 0.152: -21.6,71 -21.8,71
S$2546
  Bottom 0.152: -21.8,71 -22.8,72
S$2547
  Bottom 0.152: -23.6,71 -24.4,71.8
S$2548
  Bottom 0.152: -24.4,71.8 -24.4,72
S$2549
  Bottom 0.152: 0.4,71 1,71
S$2550
  Bottom 0.152: 1,71 2,72
S$2551
  Bottom 0.152: 2.4,71 2.6,71
S$2552
  Bottom 0.152: 2.6,71 3.6,72
S$2553
  Bottom 0.152: 4.4,71 5.2,71.8
S$2554
  Bottom 0.152: 5.2,71.8 5.2,72
S$2555
  Bottom 0.152: 6.4,71 6.8,71.4
S$2556
  Bottom 0.152: 6.8,71.4 6.8,72
S$2557
  Bottom 0.152: 8.4,71 8.4,72
S$2558
  Bottom 0.152: -1.6,71 -0.6,71
S$2559
  Bottom 0.152: -0.6,71 0.4,72
S$2560
  Bottom 0.152: -0.6,67 0.4,68
S$2561
  Bottom 0.152: 0.4,68 1.2,68
S$2562
  Bottom 0.152: 1.4,67 1.8,67
S$2563
  Bottom 0.152: 1.8,67 2.8,68
S$2564
  Bottom 0.152: 3.4,67 4.4,68
S$2565
  Bottom 0.152: 5.4,67 6,67.6
S$2566
  Bottom 0.152: 6,67.6 6,68
S$2567
  Bottom 0.152: 7.4,67 7.6,67.2
S$2568
  Bottom 0.152: 7.6,67.2 7.6,68
S$2569
  Bottom 0.152: 9.4,67 9.2,67.2
S$2570
  Bottom 0.152: 9.2,67.2 9.2,68
S$2571
  Bottom 0.152: 11.4,67 10.8,67.6
S$2572
  Bottom 0.152: 10.8,67.6 10.8,68
S$2573
  Bottom 0.152: 13.4,67 12.4,68
S$2574
  Bottom 0.152: 15.4,67 15,67
S$2575
  Bottom 0.152: 15,67 14,68
S$2576
  Bottom 0.152: 17.4,67 16.6,67
S$2577
  Bottom 0.152: 16.6,67 15.6,68
S$2578
  Bottom 0.152: 10.4,71 10,71.4
S$2579
  Bottom 0.152: 10,71.4 10,72
S$2580
  Bottom 0.152: 12.4,71 11.6,71.8
S$2581
  Bottom 0.152: 11.6,71.8 11.6,72
S$2582
  Bottom 0.152: 14.4,71 14.2,71
S$2583
  Bottom 0.152: 14.2,71 13.2,72
S$2584
  Bottom 0.152: 16.4,71 15.8,71
S$2585
  Bottom 0.152: 15.8,71 14.8,72
S$2586
  Bottom 0.152: 18.4,69 17.4,68
S$2587
  Bottom 0.152: 17.4,68 16.4,68
S$2588
  Bottom 0.152: 16.6,73 17.2,73
S$2589
  Bottom 0.152: 17.2,73 18.2,72
S$2590
  Bottom 0.152: 18.2,72 18.8,72
S$2591
  Bottom 0.152: 18.6,73 19.6,72
S$2592
  Bottom 0.152: 19.6,72 20.4,72
S$2593
  Bottom 0.152: 20.6,73 21.6,72
S$2594
  Bottom 0.152: 21.6,72 22,72
S$2595
  Bottom 0.152: 22.6,73 23.6,72
S$2596
  Bottom 0.152: 24.6,73 25.2,72.4
S$2597
  Bottom 0.152: 25.2,72.4 25.2,72
S$2598
  Bottom 0.152: 15.6,77 16.6,76
S$2599
  Bottom 0.152: 16.6,76 18,76
S$2600
  Bottom 0.152: 17.6,77 18,77
S$2601
  Bottom 0.152: 18,77 19,76
S$2602
  Bottom 0.152: 19,76 19.6,76
S$2603
  Bottom 0.152: 19.6,77 20.2,77
S$2604
  Bottom 0.152: 20.2,77 21.2,76
S$2605
  Bottom 0.152: 21.6,77 21.8,77
S$2606
  Bottom 0.152: 21.8,77 22.8,76
S$2607
  Bottom 0.152: 23.6,77 24.4,76.2
S$2608
  Bottom 0.152: 24.4,76.2 24.4,76
S$2609
  Bottom 0.152: 17.2,72 16,72
S$2610
  Bottom 0.152: 16,72 15,73
S$2611
  Bottom 0.152: 15,73 14.6,73
S$2612
  Bottom 0.152: 50.8,71 50.2,71
S$2613
  Bottom 0.152: 50.2,71 49.2,72
S$2614
  Bottom 0.152: 48.8,71 48.6,71
S$2615
  Bottom 0.152: 48.6,71 47.6,72
S$2616
  Bottom 0.152: 46.8,71 46,71.8
S$2617
  Bottom 0.152: 46,71.8 46,72
S$2618
  Bottom 0.152: 44.8,71 44.4,71.4
S$2619
  Bottom 0.152: 44.4,71.4 44.4,72
S$2620
  Bottom 0.152: 42.8,71 42.8,72
S$2621
  Bottom 0.152: 52.8,71 51.8,71
S$2622
  Bottom 0.152: 51.8,71 50.8,72
S$2623
  Bottom 0.152: 51.8,67 50.8,68
S$2624
  Bottom 0.152: 50.8,68 50,68
S$2625
  Bottom 0.152: 49.8,67 49.4,67
S$2626
  Bottom 0.152: 49.4,67 48.4,68
S$2627
  Bottom 0.152: 47.8,67 46.8,68
S$2628
  Bottom 0.152: 45.8,67 45.2,67.6
S$2629
  Bottom 0.152: 45.2,67.6 45.2,68
S$2630
  Bottom 0.152: 43.8,67 43.6,67.2
S$2631
  Bottom 0.152: 43.6,67.2 43.6,68
S$2632
  Bottom 0.152: 41.8,67 42,67.2
S$2633
  Bottom 0.152: 42,67.2 42,68
S$2634
  Bottom 0.152: 39.8,67 40.4,67.6
S$2635
  Bottom 0.152: 40.4,67.6 40.4,68
S$2636
  Bottom 0.152: 37.8,67 38.8,68
S$2637
  Bottom 0.152: 35.8,67 36.2,67
S$2638
  Bottom 0.152: 36.2,67 37.2,68
S$2639
  Bottom 0.152: 33.8,67 34.6,67
S$2640
  Bottom 0.152: 34.6,67 35.6,68
S$2641
  Bottom 0.152: 40.8,71 41.2,71.4
S$2642
  Bottom 0.152: 41.2,71.4 41.2,72
S$2643
  Bottom 0.152: 38.8,71 39.6,71.8
S$2644
  Bottom 0.152: 39.6,71.8 39.6,72
S$2645
  Bottom 0.152: 36.8,71 37,71
S$2646
  Bottom 0.152: 37,71 38,72
S$2647
  Bottom 0.152: 34.8,71 35.4,71
S$2648
  Bottom 0.152: 35.4,71 36.4,72
S$2649
  Bottom 0.152: 32.8,69 33.8,68
S$2650
  Bottom 0.152: 33.8,68 34.8,68
S$2651
  Bottom 0.152: 34.6,73 34,73
S$2652
  Bottom 0.152: 34,73 33,72
S$2653
  Bottom 0.152: 33,72 32.4,72
S$2654
  Bottom 0.152: 32.6,73 31.6,72
S$2655
  Bottom 0.152: 31.6,72 30.8,72
S$2656
  Bottom 0.152: 30.6,73 29.6,72
S$2657
  Bottom 0.152: 29.6,72 29.2,72
S$2658
  Bottom 0.152: 28.6,73 27.6,72
S$2659
  Bottom 0.152: 26.6,73 26,72.4
S$2660
  Bottom 0.152: 26,72.4 26,72
S$2661
  Bottom 0.152: 35.6,77 34.6,76
S$2662
  Bottom 0.152: 34.6,76 33.2,76
S$2663
  Bottom 0.152: 33.6,77 33.2,77
S$2664
  Bottom 0.152: 33.2,77 32.2,76
S$2665
  Bottom 0.152: 32.2,76 31.6,76
S$2666
  Bottom 0.152: 31.6,77 31,77
S$2667
  Bottom 0.152: 31,77 30,76
S$2668
  Bottom 0.152: 29.6,77 29.4,77
S$2669
  Bottom 0.152: 29.4,77 28.4,76
S$2670
  Bottom 0.152: 27.6,77 26.8,76.2
S$2671
  Bottom 0.152: 26.8,76.2 26.8,76
S$2672
  Bottom 0.152: 34,72 35.2,72
S$2673
  Bottom 0.152: 35.2,72 36.2,73
S$2674
  Bottom 0.152: 36.2,73 36.6,73
S$2675  (2 unrouted)
  Top 0.813: 65,76.5 65,67.5
  Top 1.8: 66,73.5 64,73.5 | 66,76.5 65,76.5 64,76.5 | 66,70.5 64,70.5 | 66,67.5 65,67.5 64,67.5
S$2676
  Top 1.778: -104.08,68.83 -104.08,70.35
S$2677
  Top 1.778: -104.08,73.65 -104.08,75.17
S$2678
  Top 1.778: -99,68.83 -99,70.35
S$2679
  Top 1.778: -99,73.65 -99,75.17
S$2680
  Top 1.778: -93.92,68.83 -93.92,70.35
S$2681
  Top 1.778: -93.92,73.65 -93.92,75.17
S$2682
  Top 1.778: 93.92,68.83 93.92,70.35
S$2683
  Top 1.778: 93.92,73.65 93.92,75.17
S$2684
  Top 1.778: 99,68.83 99,70.35
S$2685
  Top 1.778: 99,73.65 99,75.17
S$2686
  Top 1.778: 104.08,68.83 104.08,70.35
S$2687
  Top 1.778: 104.08,73.65 104.08,75.17
S$2696
  Bottom 0.8: 9.4,84.9 9.4,83.1
S$2697
  Bottom 0.8: 11.4,84.9 11.4,83.1
S$2698
  Bottom 0.8: 8.4,87.1 8.4,88.9
S$2699
  Bottom 0.8: 10.4,87.1 10.4,88.9
S$2700
  Bottom 0.8: 5.4,84.9 5.4,83.1
S$2701
  Bottom 0.8: 7.4,84.9 7.4,83.1
S$2702
  Bottom 0.8: 6.4,87.1 6.4,88.9
S$2703
  Bottom 0.8: 4.4,87.1 4.4,88.9
S$2704
  Bottom 0.8: 3.4,84.9 3.4,83.1
S$2705
  Bottom 0.8: 1.4,84.9 1.4,83.1
S$2706
  Bottom 0.8: 2.4,87.1 2.4,88.9
S$2707
  Bottom 0.8: 0.4,87.1 0.4,88.9
S$2708
  Bottom 0.8: -0.6,84.9 -0.6,83.1
S$2709
  Bottom 0.8: -2.6,84.9 -2.6,83.1
S$2710
  Bottom 0.8: -1.6,87.1 -1.6,88.9
S$2711
  Bottom 0.8: 17.4,84.9 17.4,83.1
S$2712
  Bottom 0.8: 19.4,84.9 19.4,83.1
S$2713
  Bottom 0.8: 16.4,87.1 16.4,88.9
S$2714
  Bottom 0.8: 18.4,87.1 18.4,88.9
S$2715
  Bottom 0.8: 13.4,84.9 13.4,83.1
S$2716
  Bottom 0.8: 15.4,84.9 15.4,83.1
S$2717
  Bottom 0.8: 12.4,87.1 12.4,88.9
S$2718
  Bottom 0.8: 14.4,87.1 14.4,88.9
S$2719
  Bottom 0.8: -7.4,92.9 -7.4,91.1
S$2720
  Bottom 0.8: -5.4,92.9 -5.4,91.1
S$2721
  Bottom 0.8: -8.4,95.1 -8.4,96.9
S$2722
  Bottom 0.8: -6.4,95.1 -6.4,96.9
S$2723
  Bottom 0.8: -11.4,92.9 -11.4,91.1
S$2724
  Bottom 0.8: -9.4,92.9 -9.4,91.1
S$2725
  Bottom 0.8: -10.4,95.1 -10.4,96.9
S$2726
  Bottom 0.8: -12.4,95.1 -12.4,96.9
S$2727
  Bottom 0.8: -13.4,92.9 -13.4,91.1
S$2728
  Bottom 0.8: -15.4,92.9 -15.4,91.1
S$2729
  Bottom 0.8: -14.4,95.1 -14.4,96.9
S$2730
  Bottom 0.8: -16.4,95.1 -16.4,96.9
S$2731
  Bottom 0.8: -17.4,92.9 -17.4,91.1
S$2732
  Bottom 0.8: -19.4,92.9 -19.4,91.1
S$2733
  Bottom 0.8: -18.4,95.1 -18.4,96.9
S$2734
  Bottom 0.8: 0.6,92.9 0.6,91.1
S$2735
  Bottom 0.8: 2.6,92.9 2.6,91.1
S$2736
  Bottom 0.8: -0.4,95.1 -0.4,96.9
S$2737
  Bottom 0.8: 1.6,95.1 1.6,96.9
S$2738
  Bottom 0.8: -3.4,92.9 -3.4,91.1
S$2739
  Bottom 0.8: -1.4,92.9 -1.4,91.1
S$2740
  Bottom 0.8: -4.4,95.1 -4.4,96.9
S$2741
  Bottom 0.8: -2.4,95.1 -2.4,96.9
S$2742
  Bottom 0.8: -24.6,84.9 -24.6,83.1
S$2743
  Bottom 0.8: -22.6,84.9 -22.6,83.1
S$2744
  Bottom 0.8: -25.6,87.1 -25.6,88.9
S$2745
  Bottom 0.8: -23.6,87.1 -23.6,88.9
S$2746
  Bottom 0.8: -28.6,84.9 -28.6,83.1
S$2747
  Bottom 0.8: -26.6,84.9 -26.6,83.1
S$2748
  Bottom 0.8: -27.6,87.1 -27.6,88.9
S$2749
  Bottom 0.8: -29.6,87.1 -29.6,88.9
S$2750
  Bottom 0.8: -30.6,84.9 -30.6,83.1
S$2751
  Bottom 0.8: -32.6,84.9 -32.6,83.1
S$2752
  Bottom 0.8: -31.6,87.1 -31.6,88.9
S$2753
  Bottom 0.8: -33.6,87.1 -33.6,88.9
S$2754
  Bottom 0.8: -34.6,84.9 -34.6,83.1
S$2755
  Bottom 0.8: -36.6,84.9 -36.6,83.1
S$2756
  Bottom 0.8: -35.6,87.1 -35.6,88.9
S$2757
  Bottom 0.8: -16.6,84.9 -16.6,83.1
S$2758
  Bottom 0.8: -14.6,84.9 -14.6,83.1
S$2759
  Bottom 0.8: -17.6,87.1 -17.6,88.9
S$2760
  Bottom 0.8: -15.6,87.1 -15.6,88.9
S$2761
  Bottom 0.8: -20.6,84.9 -20.6,83.1
S$2762
  Bottom 0.8: -18.6,84.9 -18.6,83.1
S$2763
  Bottom 0.8: -21.6,87.1 -21.6,88.9
S$2764
  Bottom 0.8: -19.6,87.1 -19.6,88.9
S$2765
  Bottom 0.8: 26.6,92.9 26.6,91.1
S$2766
  Bottom 0.8: 28.6,92.9 28.6,91.1
S$2767
  Bottom 0.8: 25.6,95.1 25.6,96.9
S$2768
  Bottom 0.8: 27.6,95.1 27.6,96.9
S$2769
  Bottom 0.8: 22.6,92.9 22.6,91.1
S$2770
  Bottom 0.8: 24.6,92.9 24.6,91.1
S$2771
  Bottom 0.8: 23.6,95.1 23.6,96.9
S$2772
  Bottom 0.8: 21.6,95.1 21.6,96.9
S$2773
  Bottom 0.8: 20.6,92.9 20.6,91.1
S$2774
  Bottom 0.8: 18.6,92.9 18.6,91.1
S$2775
  Bottom 0.8: 19.6,95.1 19.6,96.9
S$2776
  Bottom 0.8: 17.6,95.1 17.6,96.9
S$2777
  Bottom 0.8: 16.6,92.9 16.6,91.1
S$2778
  Bottom 0.8: 14.6,92.9 14.6,91.1
S$2779
  Bottom 0.8: 15.6,95.1 15.6,96.9
S$2780
  Bottom 0.8: 34.6,92.9 34.6,91.1
S$2781
  Bottom 0.8: 36.6,92.9 36.6,91.1
S$2782
  Bottom 0.8: 33.6,95.1 33.6,96.9
S$2783
  Bottom 0.8: 35.6,95.1 35.6,96.9
S$2784
  Bottom 0.8: 30.6,92.9 30.6,91.1
S$2785
  Bottom 0.8: 32.6,92.9 32.6,91.1
S$2786
  Bottom 0.8: 29.6,95.1 29.6,96.9
S$2787
  Bottom 0.8: 31.6,95.1 31.6,96.9
S$2788
  Bottom 0.8: -41.8,92.9 -41.8,91.1
S$2789
  Bottom 0.8: -39.8,92.9 -39.8,91.1
S$2790
  Bottom 0.8: -42.8,95.1 -42.8,96.9
S$2791
  Bottom 0.8: -40.8,95.1 -40.8,96.9
S$2792
  Bottom 0.8: -45.8,92.9 -45.8,91.1
S$2793
  Bottom 0.8: -43.8,92.9 -43.8,91.1
S$2794
  Bottom 0.8: -44.8,95.1 -44.8,96.9
S$2795
  Bottom 0.8: -46.8,95.1 -46.8,96.9
S$2796
  Bottom 0.8: -47.8,92.9 -47.8,91.1
S$2797
  Bottom 0.8: -49.8,92.9 -49.8,91.1
S$2798
  Bottom 0.8: -48.8,95.1 -48.8,96.9
S$2799
  Bottom 0.8: -50.8,95.1 -50.8,96.9
S$2800
  Bottom 0.8: -51.8,92.9 -51.8,91.1
S$2801
  Bottom 0.8: -53.8,92.9 -53.8,91.1
S$2802
  Bottom 0.8: -52.8,95.1 -52.8,96.9
S$2803
  Bottom 0.8: -33.8,92.9 -33.8,91.1
S$2804
  Bottom 0.8: -31.8,92.9 -31.8,91.1
S$2805
  Bottom 0.8: -34.8,95.1 -34.8,96.9
S$2806
  Bottom 0.8: -32.8,95.1 -32.8,96.9
S$2807
  Bottom 0.8: -37.8,92.9 -37.8,91.1
S$2808
  Bottom 0.8: -35.8,92.9 -35.8,91.1
S$2809
  Bottom 0.8: -38.8,95.1 -38.8,96.9
S$2810
  Bottom 0.8: -36.8,95.1 -36.8,96.9
S$2811
  Bottom 0.8: 43.8,84.9 43.8,83.1
S$2812
  Bottom 0.8: 45.8,84.9 45.8,83.1
S$2813
  Bottom 0.8: 42.8,87.1 42.8,88.9
S$2814
  Bottom 0.8: 44.8,87.1 44.8,88.9
S$2815
  Bottom 0.8: 39.8,84.9 39.8,83.1
S$2816
  Bottom 0.8: 41.8,84.9 41.8,83.1
S$2817
  Bottom 0.8: 40.8,87.1 40.8,88.9
S$2818
  Bottom 0.8: 38.8,87.1 38.8,88.9
S$2819
  Bottom 0.8: 37.8,84.9 37.8,83.1
S$2820
  Bottom 0.8: 35.8,84.9 35.8,83.1
S$2821
  Bottom 0.8: 36.8,87.1 36.8,88.9
S$2822
  Bottom 0.8: 34.8,87.1 34.8,88.9
S$2823
  Bottom 0.8: 33.8,84.9 33.8,83.1
S$2824
  Bottom 0.8: 31.8,84.9 31.8,83.1
S$2825
  Bottom 0.8: 32.8,87.1 32.8,88.9
S$2826
  Bottom 0.8: 51.8,84.9 51.8,83.1
S$2827
  Bottom 0.8: 53.8,84.9 53.8,83.1
S$2828
  Bottom 0.8: 50.8,87.1 50.8,88.9
S$2829
  Bottom 0.8: 52.8,87.1 52.8,88.9
S$2830
  Bottom 0.8: 47.8,84.9 47.8,83.1
S$2831
  Bottom 0.8: 49.8,84.9 49.8,83.1
S$2832
  Bottom 0.8: 46.8,87.1 46.8,88.9
S$2833
  Bottom 0.8: 48.8,87.1 48.8,88.9
S$2962
  Bottom 0.152: -52.8,95 -51.8,94
S$2963
  Bottom 0.152: -51.8,94 -50.8,94
S$2964
  Bottom 0.152: -50.8,95 -50.2,95
S$2965
  Bottom 0.152: -50.2,95 -49.2,94
S$2966
  Bottom 0.152: -48.8,95 -48.6,95
S$2967
  Bottom 0.152: -48.6,95 -47.6,94
S$2968
  Bottom 0.152: -46.8,95 -46,94.2
S$2969
  Bottom 0.152: -46,94.2 -46,94
S$2970
  Bottom 0.152: -44.8,95 -44.4,94.6
S$2971
  Bottom 0.152: -44.4,94.6 -44.4,94
S$2972
  Bottom 0.152: -42.8,95 -42.8,94
S$2973
  Bottom 0.152: -40.8,95 -41.2,94.6
S$2974
  Bottom 0.152: -41.2,94.6 -41.2,94
S$2975
  Bottom 0.152: -38.8,95 -39.6,94.2
S$2976
  Bottom 0.152: -39.6,94.2 -39.6,94
S$2977
  Bottom 0.152: -36.8,95 -37,95
S$2978
  Bottom 0.152: -37,95 -38,94
S$2979
  Bottom 0.152: -34.8,95 -35.4,95
S$2980
  Bottom 0.152: -35.4,95 -36.4,94
S$2981
  Bottom 0.152: -32.8,95 -33.8,94
S$2982
  Bottom 0.152: -33.8,94 -34.8,94
S$2983
  Bottom 0.152: -51.8,91 -50.8,90
S$2984
  Bottom 0.152: -50.8,90 -50,90
S$2985
  Bottom 0.152: -49.8,91 -48.8,90
S$2986
  Bottom 0.152: -48.8,90 -48.4,90
S$2987
  Bottom 0.152: -47.8,91 -46.8,90
S$2988
  Bottom 0.152: -45.8,91 -45.2,90.4
S$2989
  Bottom 0.152: -45.2,90.4 -45.2,90
S$2990
  Bottom 0.152: -43.8,91 -43.6,90.8
S$2991
  Bottom 0.152: -43.6,90.8 -43.6,90
S$2992
  Bottom 0.152: -41.8,91 -42,90.8
S$2993
  Bottom 0.152: -42,90.8 -42,90
S$2994
  Bottom 0.152: -39.8,91 -40.4,90.4
S$2995
  Bottom 0.152: -40.4,90.4 -40.4,90
S$2996
  Bottom 0.152: -37.8,91 -38.8,90
S$2997
  Bottom 0.152: -35.8,91 -36.8,90
S$2998
  Bottom 0.152: -36.8,90 -37.2,90
S$2999
  Bottom 0.152: -33.8,91 -34.8,90
S$3000
  Bottom 0.152: -34.8,90 -35.6,90
S$3001
  Bottom 0.152: -36.6,85 -35.6,86
S$3002
  Bottom 0.152: -35.6,86 -34,86
S$3003
  Bottom 0.152: -34.6,85 -33.8,85
S$3004
  Bottom 0.152: -33.8,85 -32.8,86
S$3005
  Bottom 0.152: -32.8,86 -32.4,86
S$3006
  Bottom 0.152: -32.6,85 -31.8,85
S$3007
  Bottom 0.152: -31.8,85 -30.8,86
S$3008
  Bottom 0.152: -30.6,85 -30.2,85
S$3009
  Bottom 0.152: -30.2,85 -29.2,86
S$3010
  Bottom 0.152: -28.6,85 -27.6,86
S$3011
  Bottom 0.152: -26.6,85 -26,85.6
S$3012
  Bottom 0.152: -26,85.6 -26,86
S$3013
  Bottom 0.152: -35.6,89 -35,89
S$3014
  Bottom 0.152: -35,89 -34,90
S$3015
  Bottom 0.152: -34,90 -33.2,90
S$3016
  Bottom 0.152: -33.6,89 -33,89
S$3017
  Bottom 0.152: -33,89 -32,90
S$3018
  Bottom 0.152: -32,90 -31.6,90
S$3019
  Bottom 0.152: -31.6,89 -31,89
S$3020
  Bottom 0.152: -31,89 -30,90
S$3021
  Bottom 0.152: -29.6,89 -29.4,89
S$3022
  Bottom 0.152: -29.4,89 -28.4,90
S$3023
  Bottom 0.152: -27.6,89 -26.8,89.8
S$3024
  Bottom 0.152: -26.8,89.8 -26.8,90
S$3025
  Bottom 0.152: 1.6,95 0.6,94
S$3026
  Bottom 0.152: 0.6,94 -0.4,94
S$3027
  Bottom 0.152: -0.4,95 -1,95
S$3028
  Bottom 0.152: -1,95 -2,94
S$3029
  Bottom 0.152: -2.4,95 -2.6,95
S$3030
  Bottom 0.152: -2.6,95 -3.6,94
S$3031
  Bottom 0.152: -4.4,95 -5.2,94.2
S$3032
  Bottom 0.152: -5.2,94.2 -5.2,94
S$3033
  Bottom 0.152: -6.4,95 -6.8,94.6
S$3034
  Bottom 0.152: -6.8,94.6 -6.8,94
S$3035
  Bottom 0.152: -8.4,95 -8.4,94
S$3036
  Bottom 0.152: -10.4,95 -10,94.6
S$3037
  Bottom 0.152: -10,94.6 -10,94
S$3038
  Bottom 0.152: -12.4,95 -11.6,94.2
S$3039
  Bottom 0.152: -11.6,94.2 -11.6,94
S$3040
  Bottom 0.152: -14.4,95 -14.2,95
S$3041
  Bottom 0.152: -14.2,95 -13.2,94
S$3042
  Bottom 0.152: -16.4,95 -15.8,95
S$3043
  Bottom 0.152: -15.8,95 -14.8,94
S$3044
  Bottom 0.152: -18.4,95 -17.4,94
S$3045
  Bottom 0.152: -17.4,94 -16.4,94
S$3046
  Bottom 0.152: 0.6,91 -0.4,90
S$3047
  Bottom 0.152: -0.4,90 -1.2,90
S$3048
  Bottom 0.152: -1.4,91 -2.4,90
S$3049
  Bottom 0.152: -2.4,90 -2.8,90
S$3050
  Bottom 0.152: -3.4,91 -4.4,90
S$3051
  Bottom 0.152: -5.4,91 -6,90.4
S$3052
  Bottom 0.152: -6,90.4 -6,90
S$3053
  Bottom 0.152: -7.4,91 -7.6,90.8
S$3054
  Bottom 0.152: -7.6,90.8 -7.6,90
S$3055
  Bottom 0.152: -9.4,91 -9.2,90.8
S$3056
  Bottom 0.152: -9.2,90.8 -9.2,90
S$3057
  Bottom 0.152: -11.4,91 -10.8,90.4
S$3058
  Bottom 0.152: -10.8,90.4 -10.8,90
S$3059
  Bottom 0.152: -13.4,91 -12.4,90
S$3060
  Bottom 0.152: -15.4,91 -14.4,90
S$3061
  Bottom 0.152: -14.4,90 -14,90
S$3062
  Bottom 0.152: -17.4,91 -16.4,90
S$3063
  Bottom 0.152: -16.4,90 -15.6,90
S$3064
  Bottom 0.152: -14.6,85 -15.6,86
S$3065
  Bottom 0.152: -15.6,86 -17.2,86
S$3066
  Bottom 0.152: -16.6,85 -17.4,85
S$3067
  Bottom 0.152: -17.4,85 -18.4,86
S$3068
  Bottom 0.152: -18.4,86 -18.8,86
S$3069
  Bottom 0.152: -18.6,85 -19.4,85
S$3070
  Bottom 0.152: -19.4,85 -20.4,86
S$3071
  Bottom 0.152: -20.6,85 -21,85
S$3072
  Bottom 0.152: -21,85 -22,86
S$3073
  Bottom 0.152: -22.6,85 -23.6,86
S$3074
  Bottom 0.152: -24.6,85 -25.2,85.6
S$3075
  Bottom 0.152: -25.2,85.6 -25.2,86
S$3076
  Bottom 0.152: -15.6,89 -16.2,89
S$3077
  Bottom 0.152: -16.2,89 -17.2,90
S$3078
  Bottom 0.152: -17.2,90 -18,90
S$3079
  Bottom 0.152: -17.6,89 -18.2,89
S$3080
  Bottom 0.152: -18.2,89 -19.2,90
S$3081
  Bottom 0.152: -19.2,90 -19.6,90
S$3082
  Bottom 0.152: -19.6,89 -20.2,89
S$3083
  Bottom 0.152: -20.2,89 -21.2,90
S$3084
  Bottom 0.152: -21.6,89 -21.8,89
S$3085
  Bottom 0.152: -21.8,89 -22.8,90
S$3086
  Bottom 0.152: -23.6,89 -24.4,89.8
S$3087
  Bottom 0.152: -24.4,89.8 -24.4,90
S$3088
  Bottom 0.152: 0.4,89 1,89
S$3089
  Bottom 0.152: 1,89 2,90
S$3090
  Bottom 0.152: 2.4,89 2.6,89
S$3091
  Bottom 0.152: 2.6,89 3.6,90
S$3092
  Bottom 0.152: 4.4,89 5.2,89.8
S$3093
  Bottom 0.152: 5.2,89.8 5.2,90
S$3094
  Bottom 0.152: 6.4,89 6.8,89.4
S$3095
  Bottom 0.152: 6.8,89.4 6.8,90
S$3096
  Bottom 0.152: 8.4,89 8.4,90
S$3097
  Bottom 0.152: -1.6,89 -0.6,89
S$3098
  Bottom 0.152: -0.6,89 0.4,90
S$3099
  Bottom 0.152: -0.6,85 0.4,86
S$3100
  Bottom 0.152: 0.4,86 1.2,86
S$3101
  Bottom 0.152: 1.4,85 1.8,85
S$3102
  Bottom 0.152: 1.8,85 2.8,86
S$3103
  Bottom 0.152: 3.4,85 4.4,86
S$3104
  Bottom 0.152: 5.4,85 6,85.6
S$3105
  Bottom 0.152: 6,85.6 6,86
S$3106
  Bottom 0.152: 7.4,85 7.6,85.2
S$3107
  Bottom 0.152: 7.6,85.2 7.6,86
S$3108
  Bottom 0.152: 9.4,85 9.2,85.2
S$3109
  Bottom 0.152: 9.2,85.2 9.2,86
S$3110
  Bottom 0.152: 11.4,85 10.8,85.6
S$3111
  Bottom 0.152: 10.8,85.6 10.8,86
S$3112
  Bottom 0.152: 13.4,85 12.4,86
S$3113
  Bottom 0.152: 15.4,85 15,85
S$3114
  Bottom 0.152: 15,85 14,86
S$3115
  Bottom 0.152: 17.4,85 16.6,85
S$3116
  Bottom 0.152: 16.6,85 15.6,86
S$3117
  Bottom 0.152: 10.4,89 10,89.4
S$3118
  Bottom 0.152: 10,89.4 10,90
S$3119
  Bottom 0.152: 12.4,89 11.6,89.8
S$3120
  Bottom 0.152: 11.6,89.8 11.6,90
S$3121
  Bottom 0.152: 14.4,89 14.2,89
S$3122
  Bottom 0.152: 14.2,89 13.2,90
S$3123
  Bottom 0.152: 16.4,89 15.8,89
S$3124
  Bottom 0.152: 15.8,89 14.8,90
S$3125
  Bottom 0.152: 18.4,87 17.4,86
S$3126
  Bottom 0.152: 17.4,86 16.4,86
S$3127
  Bottom 0.152: 16.6,91 17.2,91
S$3128
  Bottom 0.152: 17.2,91 18.2,90
S$3129
  Bottom 0.152: 18.2,90 18.8,90
S$3130
  Bottom 0.152: 18.6,91 19.6,90
S$3131
  Bottom 0.152: 19.6,90 20.4,90
S$3132
  Bottom 0.152: 20.6,91 21.6,90
S$3133
  Bottom 0.152: 21.6,90 22,90
S$3134
  Bottom 0.152: 22.6,91 23.6,90
S$3135
  Bottom 0.152: 24.6,91 25.2,90.4
S$3136
  Bottom 0.152: 25.2,90.4 25.2,90
S$3137
  Bottom 0.152: 15.6,95 16.6,94
S$3138
  Bottom 0.152: 16.6,94 18,94
S$3139
  Bottom 0.152: 17.6,95 18,95
S$3140
  Bottom 0.152: 18,95 19,94
S$3141
  Bottom 0.152: 19,94 19.6,94
S$3142
  Bottom 0.152: 19.6,95 20.2,95
S$3143
  Bottom 0.152: 20.2,95 21.2,94
S$3144
  Bottom 0.152: 21.6,95 21.8,95
S$3145
  Bottom 0.152: 21.8,95 22.8,94
S$3146
  Bottom 0.152: 23.6,95 24.4,94.2
S$3147
  Bottom 0.152: 24.4,94.2 24.4,94
S$3148
  Bottom 0.152: 17.2,90 16,90
S$3149
  Bottom 0.152: 16,90 15,91
S$3150
  Bottom 0.152: 15,91 14.6,91
S$3151
  Bottom 0.152: 50.8,89 50.2,89
S$3152
  Bottom 0.152: 50.2,89 49.2,90
S$3153
  Bottom 0.152: 48.8,89 48.6,89
S$3154
  Bottom 0.152: 48.6,89 47.6,90
S$3155
  Bottom 0.152: 46.8,89 46,89.8
S$3156
  Bottom 0.152: 46,89.8 46,90
S$3157
  Bottom 0.152: 44.8,89 44.4,89.4
S$3158
  Bottom 0.152: 44.4,89.4 44.4,90
S$3159
  Bottom 0.152: 42.8,89 42.8,90
S$3160
  Bottom 0.152: 52.8,89 51.8,89
S$3161
  Bottom 0.152: 51.8,89 50.8,90
S$3162
  Bottom 0.152: 51.8,85 50.8,86
S$3163
  Bottom 0.152: 50.8,86 50,86
S$3164
  Bottom 0.152: 49.8,85 49.4,85
S$3165
  Bottom 0.152: 49.4,85 48.4,86
S$3166
  Bottom 0.152: 47.8,85 46.8,86
S$3167
  Bottom 0.152: 45.8,85 45.2,85.6
S$3168
  Bottom 0.152: 45.2,85.6 45.2,86
S$3169
  Bottom 0.152: 43.8,85 43.6,85.2
S$3170
  Bottom 0.152: 43.6,85.2 43.6,86
S$3171
  Bottom 0.152: 41.8,85 42,85.2
S$3172
  Bottom 0.152: 42,85.2 42,86
S$3173
  Bottom 0.152: 39.8,85 40.4,85.6
S$3174
  Bottom 0.152: 40.4,85.6 40.4,86
S$3175
  Bottom 0.152: 37.8,85 38.8,86
S$3176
